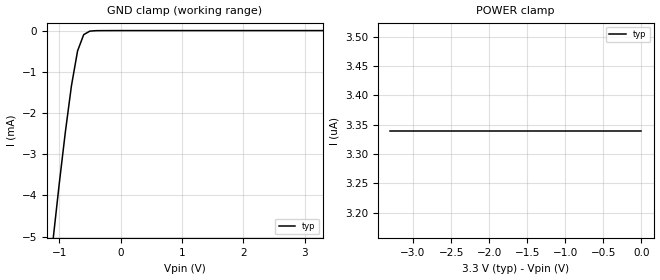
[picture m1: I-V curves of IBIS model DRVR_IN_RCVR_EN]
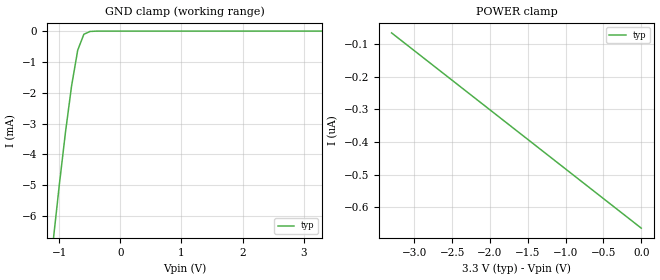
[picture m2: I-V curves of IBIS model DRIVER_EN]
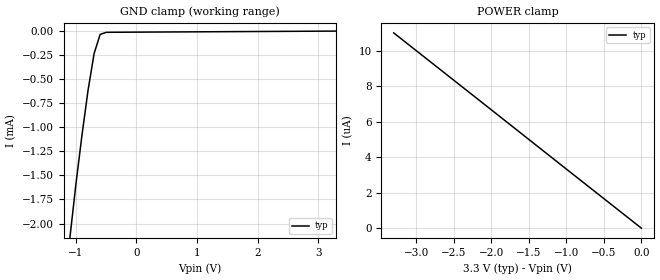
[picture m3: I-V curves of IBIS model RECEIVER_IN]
|   Texas Instruments Incorporated
|   Data Transmissions Products
|   IBIS Model for SN65LVDS050
|   16D SOIC Package
[IBIS Ver]   2.1
[Comment char]   |_char
[File name]   lvds050.ibs
[File Rev]   2.0
[Date]   25Sep98
[Source]   File originated at Texas Instruments Incorporated.
   Data Transmission Products Group.
[Notes]
[Disclaimer]
(C) Copyright Texas Instruments Incorporated 1998
   All rights reserved
  Texas Instruments Incorporated hereby grants the user of this IBIS
model a non-exclusive, nontransferable license to use this IBIS model
under the following terms.  Before using this IBIS model, the user
should read this license.  If the user does not accept these terms,
the IBIS model should be returned to Texas Instruments within 30 days.
  The user is granted this license only to use the IBIS model and
is not granted rights to sell, load, rent, lease or license the IBIS
model in whole or in part, or in modified form to anyone other than
user.  User may modify the IBIS model to suit its specific applications
but rights to derivative works and such modifications shall belong to
Texas Instruments.
  This IBIS model is provided on an "AS IS" basis and Texas Instruments
makes absolutely no warranty with respect to the information contained
herein.  TEXAS INSTRUMENTS DISCLAIMS AND CUSTOMER WAIVES ALL WARRANTIES,
EXPRESS OR IMPLIED, INCLUDING WARRANTIES OF MERCHANTABILITY OR FITNESS
FOR A PARTICULAR PURPOSE. The entire risk as to quality and performance
is with the Customer. ACCORDINGLY, IN NO EVENT SHALL THE COMPANY BE LIABLE
FOR ANY DAMAGES, WHETHER IN CONTRACT OR TORT,INCLUDING ANY LOST PROFITS
OR OTHER INCIDENTAL, CONSEQUENTIAL, EXEMPLARY, OR PUNITIVE DAMAGES ARISING
OUT OF THE USE OR APPLICATION OF THE IBIS model provided in this package.
Further, Texas Instruments reserves the right to discontinue or make changes
without notice to any product herein to improve reliability, function, or
design. Texas Instruments does not convey any license under patent rights
or any other intellectual property rights, including those of third parties.
Contact Texas Instruments at ATTN:DATA TRANSMISSIONS
Thomas Fisher 8505 Forest Lane, M/S 8710, Dallas, TX 75243-4136
[Copyright]   Copyright 1998, Texas Instruments, All Rights Reserved
[Component]   LVDS050D
[Manufacturer]  Texas Instruments Incorporated
[Package]
|   typ   min   max
R_pkg   0.035   0.030   0.040
L_pkg   2.181nH   1.231nH   3.257nH
C_pkg   0.322pF   0.163pF   0.546pF
[Pin]   signal_name   model_name   R_pin   L_pin   C_pin
1   1B   RECEIVER_IN   0.040   3.251n   0.546p
2   1A   RECEIVER_IN   0.039   2.561n   0.393p
3   1R   RECEIVER_OUT   0.030   1.681n   0.186p
4   RE   DRVR_IN_RCVR_EN  0.030   1.231n   0.163p
5   2R   RECEIVER_OUT   0.030   1.231n   0.163p
6   2A   RECEIVER_IN   0.030   1.681n   0.186p
7   2B   RECEIVER_IN   0.039   2.564n   0.393p
8   GND   GND   0.040   3.257n   0.545p
9   2D   DRVR_IN_RCVR_EN  0.040   3.247n   0.546p
10   2Y   DRIVER_OUT   0.039   2.558n   0.394p
11   2Z   DRIVER_OUT   0.030   1.681n   0.187p
12   DE   DRIVER_EN   0.030   1.231n   0.163p
13   1Z   DRIVER_OUT   0.030   1.231n   0.163p
14   1Y   DRIVER_OUT   0.030   1.681n   0.187p
15   1D   DRVR_IN_RCVR_EN  0.039   2.558n   0.394p
16   VCC   POWER   0.040   3.246n   0.546p
[Diff_pin]   inv_pin   vdiff   tdelay_typ   tdelay_min   tdelay_max
| The 'xA' pin is Diff_pin and the 'xB' pin is the inv_pin
2   1   0.100   0 0 0
6   7   0.100   0 0 0
| Models and submodels in the file (5): DRVR_IN_RCVR_EN (Input), DRIVER_EN (Input), RECEIVER_IN (Input), DRIVER_OUT (3-state), RECEIVER_OUT (3-state)
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|   Driver Input/Receiver Enable MODEL
[Model]   DRVR_IN_RCVR_EN
Model_type   Input
|Signals   RE,2D,1D
Vinh = 2.0
Vinl = 0.8
|   typ   min   max
C_comp   1.0pF   NA   NA
|   typ   min   max
[Temperature Range]   25.0   NA   NA
[Voltage range]   3.3V   3.0V   3.6V
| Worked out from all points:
|   GND clamp passes 1 mA (typ) near -0.76 V on its own axis
[GND_clamp]
|   Voltage   I(typ)   I(min)   I(max)
-3.3V     -43.1mA    NA         NA
-1.1V     -5.08mA    NA         NA
-1V       -3.73mA    NA         NA
-900mV    -2.47mA    NA         NA
-800mV    -1.34mA    NA         NA
-700mV    -493uA     NA         NA
-600mV    -98.5uA    NA         NA
-500mV    -13.3uA    NA         NA
3.3V      3.34pA     NA         NA
[Power_clamp]
| Note that the[POWER_clamp]voltage table is referenced to Vcc
| and is calculated using Vtable=Vcc - Vmeasured.
|   Voltage   I(typ)   I(min)   I(max)
-3.3V     3.34uA     NA         NA
-2.7V     3.34uA     NA         NA
-2V       3.34uA     NA         NA
-800mV    3.34uA     NA         NA
0V        3.34uA     NA         NA
|   Driver Enable  MODEL
[Model]   DRIVER_EN
Model_type   Input
|Signals   DE
Vinh = 2.0
Vinl = 0.8
|   typ   min   max
C_comp   1.0pF   NA   NA
|   typ   min   max
[Temperature Range]   25.0   NA   NA
[Voltage range]   3.3V   3.0V   3.6V
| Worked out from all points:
|   GND clamp passes 1 mA (typ) near -0.73 V on its own axis
[GND_clamp]
|   Voltage   I(typ)   I(min)   I(max)
-3.3V     -61.4mA    NA         NA
-1.1V     -6.77mA    NA         NA
-1V       -4.96mA    NA         NA
-900mV    -3.27mA    NA         NA
-800mV    -1.77mA    NA         NA
-700mV    -618uA     NA         NA
-600mV    -105uA     NA         NA
-500mV    -12.4uA    NA         NA
-400mV    -1.61uA    NA         NA
3.3V      0A         NA         NA
[Power_clamp]
| Note that the[POWER_clamp]voltage table is referenced to Vcc
| and is calculated using Vtable=Vcc - Vmeasured.
|   Voltage   I(typ)   I(min)   I(max)
-3.3V     -66.4nA    NA         NA
0V        -664nA     NA         NA
|   Receiver Input MODEL
[Model]   RECEIVER_IN
Model_type   Input
|Signals   1A,1B,2A,2B
Vinh = 2.0
Vinl = 0.8
|   typ   min   max
C_comp   1.0pF   NA   NA
|   typ   min   max
[Temperature Range]   25.0   NA   NA
[Voltage range]   3.3V   3.0V   3.6V
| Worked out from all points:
|   GND clamp passes 1 mA (typ) near -0.88 V on its own axis
[GND_clamp]
|   Voltage   I(typ)   I(min)   I(max)
-3.3V     -22.5mA    NA         NA
-1.1V     -2.15mA    NA         NA
-1V       -1.59mA    NA         NA
-900mV    -1.08mA    NA         NA
-800mV    -616uA     NA         NA
-700mV    -234uA     NA         NA
-600mV    -34.5uA    NA         NA
-500mV    -13.2uA    NA         NA
-400mV    -12.3uA    NA         NA
3.3V      444pA      NA         NA
[Power_clamp]
| Note that the[POWER_clamp]voltage table is referenced to Vcc
| and is calculated using Vtable=Vcc - Vmeasured.
|   Voltage   I(typ)   I(min)   I(max)
-3.3V     11uA       NA         NA
-2V       6.67uA     NA         NA
-1V       3.33uA     NA         NA
0V        0A         NA         NA
